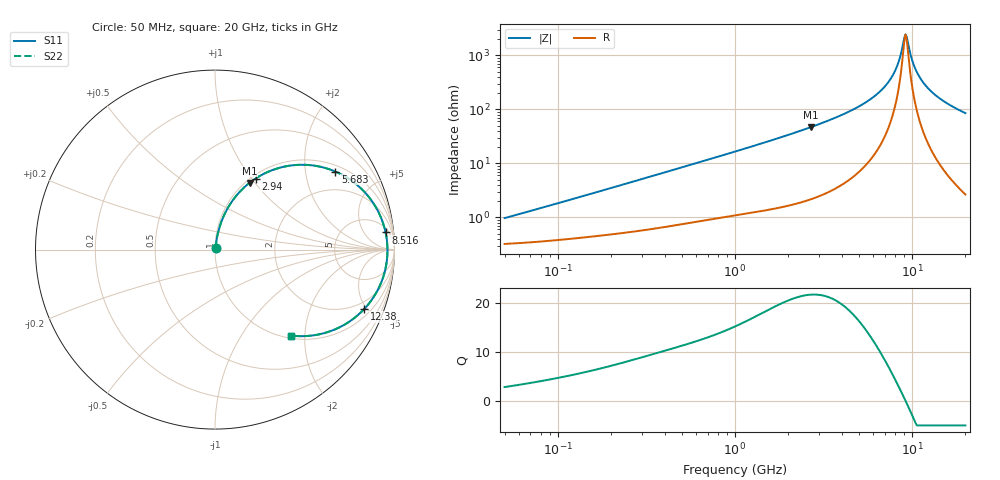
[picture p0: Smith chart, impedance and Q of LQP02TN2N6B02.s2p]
!Murata Part Number: LQP02TN2N6B02
!These Parameters are Measured in Series Mode Connection
!  o--[Z]--o
!Port1  Port2
!  o-------o
!Freq. Start=50[MHz] Stop=20[GHz], 401[Steps]
# Hz S RI R 50
!Freq.(Hz) S11(Real) S11(Imag) S21(Real) S21(Imag) S12(Real) S12(Imag) S22(Real) S22(Imag)
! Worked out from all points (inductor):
!   401 points, 50 MHz to 20 GHz, reference 50 ohm
!   read as one part in series: L = 2.88 nH near 53.89 MHz
!   highest Q = 21.7 at 2.687 GHz (marker M1), where L = 2.79 nH
!   self-resonance near 9.178 GHz
!   S11 on the Smith chart (normalised r, x): 50 MHz: 1.01, +0.02; 2.94 GHz: 1.05, +1.05; 5.683 GHz: 1.21, +2.92; 8.516 GHz: 8, +17; 12.38 GHz: 1.45, -4.81; 20 GHz: 1.05, -1.71
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5e7  0.00328 0.00907  0.9967 -0.00907  0.9967 -0.00907  0.00328 0.00907
1.364002e8  0.00474 0.0238  0.9953 -0.0238  0.9953 -0.0238  0.00474 0.0238
3.721004e8  0.0102 0.062  0.9898 -0.062  0.9898 -0.062  0.0102 0.062
1e9  0.0364 0.1573  0.9636 -0.1573  0.9636 -0.1573  0.0364 0.1573
1.766834e9  0.0916 0.2641  0.9084 -0.2641  0.9084 -0.2641  0.0916 0.2641
2.687447e9  0.1923 0.3718  0.8077 -0.3718  0.8077 -0.3718  0.1923 0.3718
2.728004e9  0.1976 0.3758  0.8024 -0.3758  0.8024 -0.3758  0.1976 0.3758
2.940159e9  0.226 0.3958  0.774 -0.3958  0.774 -0.3958  0.226 0.3958
4.34015e9  0.4458 0.4711  0.5542 -0.4711  0.5542 -0.4711  0.4458 0.4711
5.683258e9  0.6708 0.4349  0.3292 -0.4349  0.3292 -0.4349  0.6708 0.4349
6.601595e9  0.8015 0.3521  0.1985 -0.3521  0.1985 -0.3521  0.8015 0.3521
7.442007e9  0.8895 0.2473  0.1105 -0.2473  0.1105 -0.2473  0.8895 0.2473
8.020766e9  0.9295 0.1663  0.0705 -0.1663  0.0705 -0.1663  0.9295 0.1663
8.516016e9  0.9505 0.0953  0.0495 -0.0953  0.0495 -0.0953  0.9505 0.0953
9.041845e9  0.9603 0.021  0.0397 -0.021  0.0397 -0.021  0.9603 0.021
9.316812e9  0.9608 -0.0167  0.0392 0.0167  0.0392 0.0167  0.9608 -0.0167
1.004137e10  0.949 -0.1098  0.051 0.1098  0.051 0.1098  0.949 -0.1098
1.050288e10  0.9335 -0.1634  0.0665 0.1634  0.0665 0.1634  0.9335 -0.1634
1.131968e10  0.895 -0.246  0.105 0.246  0.105 0.246  0.895 -0.246
1.238412e10  0.8322 -0.3303  0.1678 0.3303  0.1678 0.3303  0.8322 -0.3303
1.550395e10  0.6359 -0.4569  0.3641 0.4569  0.3641 0.4569  0.6359 -0.4569
2e10  0.4245 -0.479  0.5755 0.479  0.5755 0.479  0.4245 -0.479
